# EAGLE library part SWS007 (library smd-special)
SMD Dip Switch 7 pol.
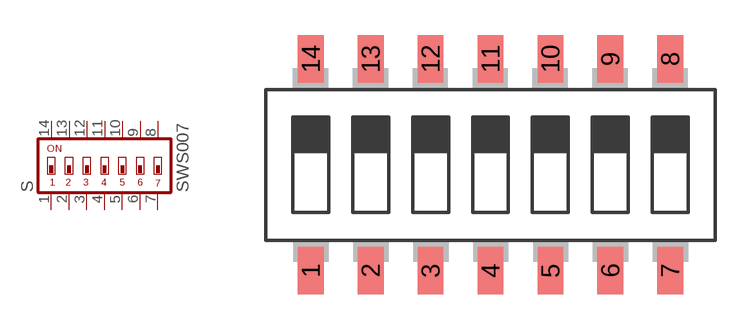
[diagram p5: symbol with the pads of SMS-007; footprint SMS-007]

Designator prefix S

## SWS007  [SMS-007]
1  1  pas
2  2  pas
3  3  pas
4  4  pas
5  5  pas
6  6  pas
7  7  pas
8  8  pas
9  9  pas
10  10  pas
11  11  pas
12  12  pas
13  13  pas
14  14  pas

## Footprint SMS-007 (pad centres in mm)
DIP SWITCH
smd 1.092 x 2.007: 1 -7.62,-4.496; 2 -5.08,-4.496; 3 -2.54,-4.496; 4 0,-4.496; 5 2.54,-4.496; 6 5.08,-4.496; 7 7.62,-4.496; 8 7.62,4.496; 9 5.08,4.496; 10 2.54,4.496; 11 0,4.496; 12 -2.54,4.496; 13 -5.08,4.496; 14 -7.62,4.496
